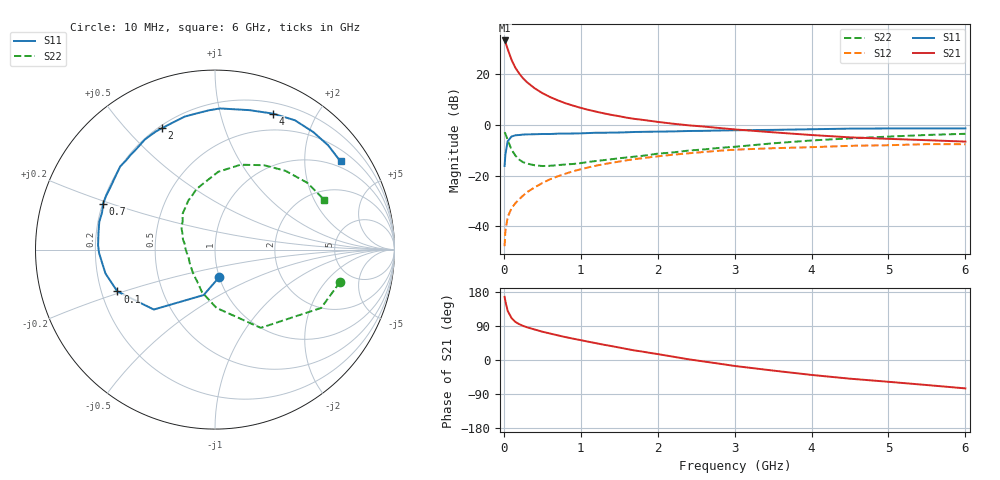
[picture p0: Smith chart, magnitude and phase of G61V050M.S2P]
! SIEMENS Small Signal Semiconductors
! BFG193
! Si NPN RF Bipolar Junction Transistor in SOT223
! VCE = 1 V  IC = 50 mA
! Common Emitter S-Parameters:  August  1996
# GHz  S  MA  R  50
!  f  S11  S21  S12  S22
! GHz  MAG  ANG  MAG  ANG  MAG  ANG  MAG  ANG
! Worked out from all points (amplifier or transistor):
!   36 points, 10 MHz to 6 GHz, reference 50 ohm
!   highest |S21| = 33.5 dB at 10 MHz (marker M1)
!   |S21| within 3 dB of that: start of sweep to 45.59 MHz
!   unconditionally stable (mu >= 1): start of sweep to 13.29 MHz; 218.6 MHz to end of sweep
!   at 250 MHz: K = 1.03, MAG = 22.2 dB, |S12| = -28.0 dB
!   at 1.4 GHz: K = 1.13, MAG = 7.3 dB, |S12| = -15.0 dB
!   at 6 GHz: K = 1.03, MAG = -0.5 dB, |S12| = -7.6 dB
!   S11 on the Smith chart (normalised r, x): 10 MHz: 1.00, -0.31; 100 MHz: 0.27, -0.19; 700 MHz: 0.20, +0.19; 2 GHz: 0.21, +0.63; 4 GHz: 0.31, +1.47; 6 GHz: 0.81, +2.96
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0.01  0.1546 -81.0  47.05 166.6  0.004 77.0  0.7194 -14.6
0.02  0.2609 -104.0  43.81 155.1  0.008 71.3  0.6747 -28.8
0.05  0.4773 -135.6  31.77 129.6  0.0151 59.7  0.5049 -59.7
0.1  0.592 -156.8  19.48 110.7  0.0225 56.2  0.3252 -88.5
0.15  0.6245 -167.7  13.55 100.4  0.0284 58.1  0.2485 -106.9
0.2  0.6337 -173.5  10.43 94.6  0.0339 60.9  0.2063 -118.1
0.25  0.6461 -178.3  8.382 90.0  0.04 62.6  0.1836 -130.1
0.3  0.6518 177.9  7.039 86.4  0.0466 63.9  0.1727 -137.7
0.4  0.6558 172.0  5.333 80.5  0.0582 64.5  0.1595 -151.8
0.5  0.663 166.5  4.279 74.7  0.0708 63.7  0.1541 -162.2
0.6  0.6623 161.9  3.577 69.9  0.0841 62.8  0.1557 -169.6
0.7  0.6736 157.7  3.081 65.1  0.0963 61.3  0.1604 -176.2
0.9  0.6784 149.3  2.415 56.3  0.1217 57.3  0.1692 171.3
1.1  0.6923 142.2  1.988 48.2  0.1448 53.3  0.1858 163.2
1.6  0.7176 125.5  1.393 28.9  0.2004 41.2  0.2281 144.1
2  0.7381 113.6  1.151 15.6  0.2393 31.4  0.2709 131.5
2.2  0.7463 108.1  1.06 8.8  0.2583 26.4  0.2863 125.3
3.5  0.8001 76.2  0.716 -27.9  0.347 -6.6  0.4339 87.6
4  0.8237 66.9  0.633 -39.4  0.3636 -16.2  0.494 73.2
4.5  0.847 58.3  0.569 -49.3  0.3872 -26.1  0.5435 59.9
5.5  0.8573 42.7  0.5 -66.1  0.4175 -48.5  0.6348 35.9
6  0.8547 35.1  0.469 -74.9  0.4156 -61.2  0.6692 24.4
